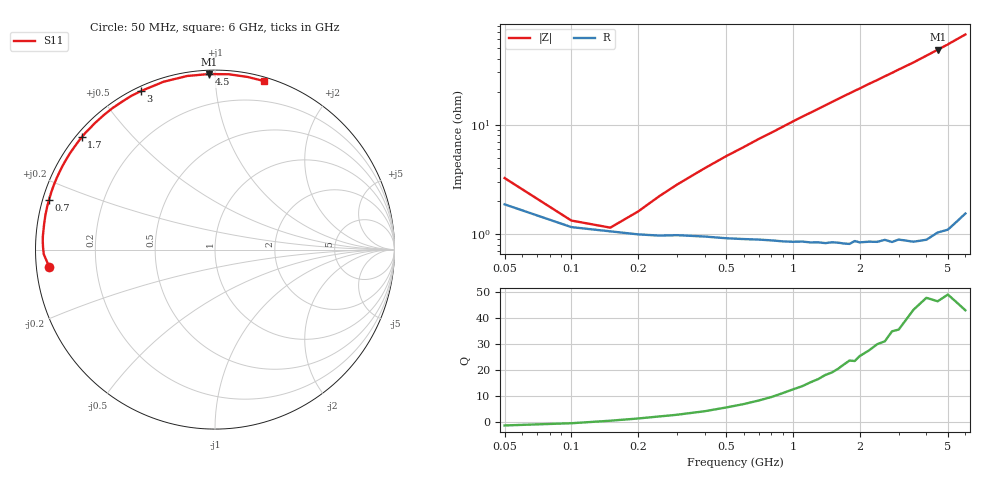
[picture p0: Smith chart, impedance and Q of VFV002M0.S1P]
! Infineon Technologies  Discrete & RF Semiconductors
! BBY 58-03
! Si Tuning Diode in SOD323
! VR =
! S-Parameters:  June  1999
# GHz  S  MA  R  50
!  f  S11
! GHz  MAG  ANG
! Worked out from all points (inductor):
!   34 points, 50 MHz to 6 GHz, reference 50 ohm
!   read as one part to ground: L = 1.63 nH near 400 MHz
!   highest Q = 47.9 at 4.5 GHz (marker M1), where L = 1.71 nH
!   S11 on the Smith chart (normalised r, x): 50 MHz: 0.04, -0.05; 700 MHz: 0.02, +0.15; 1.7 GHz: 0.02, +0.36; 3 GHz: 0.02, +0.64; 4.5 GHz: 0.02, +0.97; 6 GHz: 0.03, +1.33
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0.05  0.928 -173.9
0.1  0.9546 -178.5
0.15  0.9584 179.0
0.2  0.9609 177.1
0.25  0.962 175.4
0.4  0.9629 171.1
0.5  0.9643 168.4
0.6  0.9651 165.9
0.7  0.9656 163.3
0.8  0.9664 160.9
1  0.9679 155.9
1.1  0.9681 153.5
1.4  0.97 146.6
1.6  0.9705 142.1
1.7  0.9714 139.9
1.8  0.972 137.8
2  0.9719 133.7
2.2  0.9724 129.6
2.4  0.9734 125.9
2.6  0.9732 122.1
2.8  0.9752 118.6
3  0.9749 115.0
3.5  0.9782 107.0
4  0.9796 99.1
4.5  0.9788 92.0
5  0.9799 85.5
5.5  0.9789 79.3
6  0.978 73.8
